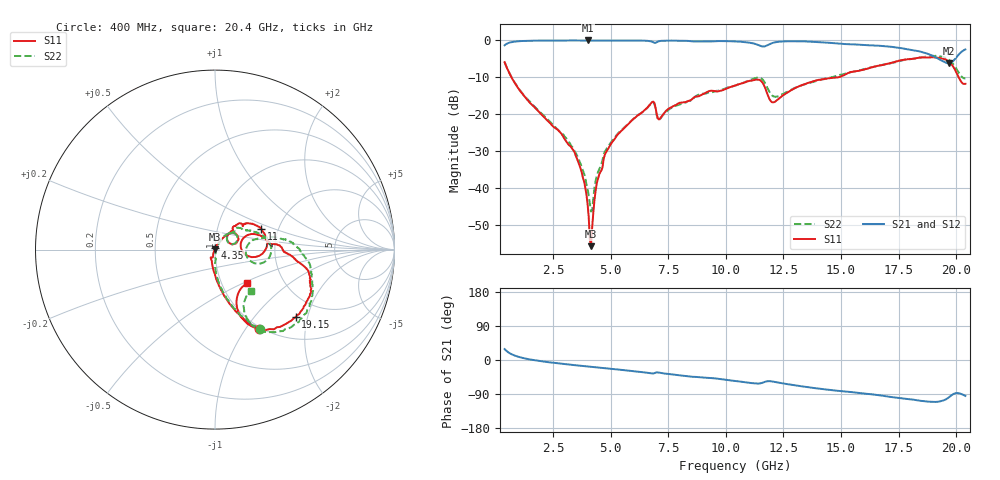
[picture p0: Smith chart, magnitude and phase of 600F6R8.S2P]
!  American Technical Ceramics  Date:  11/23/05
!  One Norden Lane
!  Huntington Station,  NY.  11746-2102
!  Tel:  (631) 622-4700  Fax:  (631) 622-4748
!  Part Number  600F6R8  Mounting Orientation: Horizontal
!  Description: Ultra Low ESR Microwave capacitors
!  Application: Coupling, Bypass, Tuning, DC Block
!  Filters, Matching
# GHZ S DB R 50
! Freq  |S11|  S11 Ph  |S21|  S21 Ph  |S12|  S12 Ph  |S22|  S22 Ph
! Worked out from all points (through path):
!   401 points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, 400 MHz to 20.4 GHz, reference 50 ohm
!   highest |S21| = 0.00 dB at 4 GHz (marker M1); lowest = -6.2 dB at 19.7 GHz (marker M2)
!   group delay of S21, straight-line fit = 16.5 ps
!   lowest |S11| = -55.8 dB at 4.15 GHz (marker M3), VSWR 1.00, Z = 49.9 + j0.136 ohm
!   |S11| at or under -10 dB: 697.6 MHz to 14.88 GHz (14.18 GHz wide, 182 % of centre); 20.11 GHz to end of sweep
!   |S22| runs from -46.4 to -4.2 dB; largest |S21 - S12| = 0.0073
!   S11 on the Smith chart (normalised r, x): 400 MHz: 0.97, -1.16; 4.35 GHz: 1.00, +0.02; 11 GHz: 1.63, +0.41; 19.15 GHz: 1.47, -1.69; 20.4 GHz: 1.31, -0.53
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0.4  -5.89 -61.0  -1.31 28.8  -1.31 28.7  -5.92 -60.6
1.2  -14.72 -85.5  -0.14 5.2  -0.15 5.1  -14.58 -83.3
2.85  -25.20 -115.5  -0.03 -9.7  -0.03 -9.8  -25.08 -85.4
3.4  -29.92 -109.4  -0.01 -13.3  -0.01 -13.3  -29.55 -87.0
3.75  -35.90 -115.6  -0.01 -15.6  0.00 -15.6  -34.46 -80.8
4  -44.33 -126.8  0.00 -17.1  -0.01 -17.2  -40.18 -63.6
4.15  -55.83 122.6  -0.01 -18.0  -0.01 -18.1  -46.43 -21.8
4.35  -40.84 74.5  -0.01 -19.2  -0.01 -19.2  -38.10 44.9
4.8  -30.39 65.7  -0.01 -21.9  -0.01 -21.9  -29.69 57.1
5.35  -25.25 57.9  -0.01 -25.4  -0.01 -25.4  -25.03 58.7
6.8  -16.71 37.4  -0.34 -35.5  -0.34 -35.5  -16.87 37.9
7.1  -21.45 32.3  -0.21 -33.2  -0.22 -33.3  -21.64 33.7
8.85  -15.10 49.0  -0.28 -45.3  -0.28 -45.2  -14.59 40.4
10.4  -12.26 36.4  -0.27 -55.4  -0.27 -55.2  -12.26 23.8
11  -11.01 24.4  -0.57 -60.0  -0.59 -60.1  -10.85 14.6
11.5  -10.85 2.0  -1.46 -61.6  -1.47 -61.6  -10.15 -5.0
12.05  -16.81 7.0  -0.63 -57.0  -0.64 -57.0  -15.12 -8.9
13.75  -11.18 14.8  -0.37 -73.2  -0.35 -73.3  -11.31 13.8
17.1  -6.20 -9.6  -1.68 -96.9  -1.68 -96.9  -6.24 -2.5
19.15  -4.64 -40.0  -4.71 -110.4  -4.73 -110.5  -4.23 -39.0
19.7  -5.85 -60.0  -6.22 -97.6  -6.19 -97.7  -5.28 -57.9
20.4  -11.77 -46.8  -2.44 -94.8  -2.44 -94.8  -10.30 -49.2
